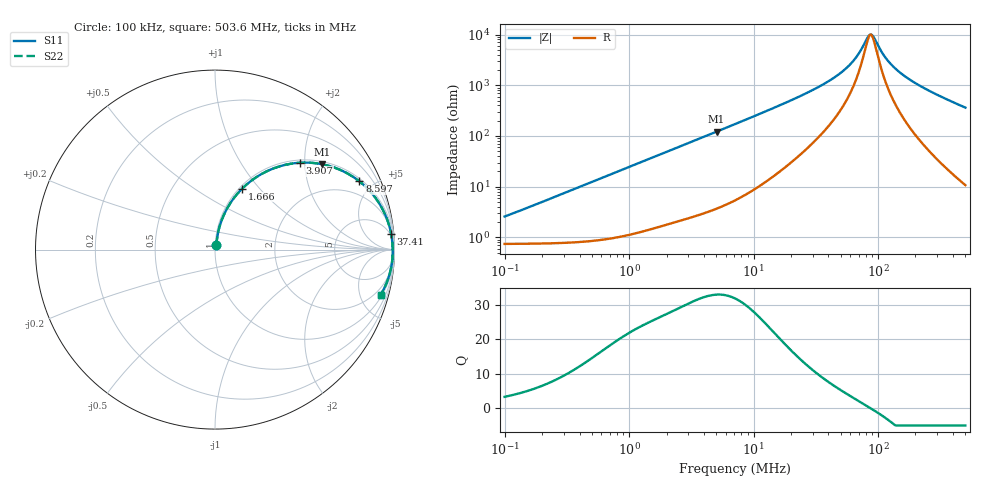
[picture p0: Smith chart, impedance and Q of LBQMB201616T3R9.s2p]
! LBQMB201616T3R9  S-PARAMETER MODEL  ( General Type )
! Model Generated by TAIYO YUDEN Corporation (http://www.ty-top.com)
! Version 1.0
! TAIYO YUDEN Control No. 191025NI43SB-FBB
! Copyright(c) 2019 TAIYO YUDEN CO.,LTD. All Rights Reserved.
! Product Description (link to TY-COMPAS)
! https://ds.yuden.co.jp/TYCOMPAS/or/detail?pn=LBQMB201616T3R9J&u=M
! Products Name : Inductors
! Characteristics :
!  Inductance : 3.9 uH , SRF(min) : 43 MHz , DC Resistance(max) : 0.962 Ohm , Rated Current : 275 mA
!  Case Size : 2.0 x 1.6 / 0.079 x 0.063 [mm/inch] , Thickness : 1.6 / 0.063 [mm/inch]
!  (Conditions: Temperature = 25 degC , DC Bias Current/Voltage = 0A / 0V)
! External Node Assignments :
!  1  o---GGG---o  2
! GND o---------o GND
! Frequency Range : 0.1MHz  -  503.601575MHz  [ 402 STEP ]
# MHz S RI R 50
! Freq[MHz].  S11 Real  S11 Imag  S21 Real  S21 Imag  S12 Real  S12 Imag  S22 Real  S22 Imag
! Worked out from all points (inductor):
!   401 points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, 100 kHz to 503.6 MHz, reference 50 ohm
!   read as one part in series: L = 3.94 uH near 104.4 kHz
!   highest Q = 33 at 5.046 MHz (marker M1), where L = 3.84 uH
!   self-resonance near 85.88 MHz
!   S11 on the Smith chart (normalised r, x): 100 kHz: 1.01, +0.05; 1.666 MHz: 1.03, +0.81; 3.907 MHz: 1.06, +1.89; 8.597 MHz: 1.14, +4.16; 37.41 MHz: 4, +22; 503.6 MHz: 1.21, -7.25
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0.1  0.00799 0.0244  0.992 -0.0244  0.992 -0.0244  0.00799 0.0244
0.416965  0.0184 0.1003  0.9816 -0.1003  0.9816 -0.1003  0.0184 0.1003
0.937126  0.0596 0.2145  0.9404 -0.2145  0.9404 -0.2145  0.0596 0.2145
1.666053  0.1516 0.3399  0.8484 -0.3399  0.8484 -0.3399  0.1516 0.3399
1.738598  0.162 0.3499  0.838 -0.3499  0.838 -0.3499  0.162 0.3499
3.907486  0.4723 0.4839  0.5277 -0.4839  0.5277 -0.4839  0.4723 0.4839
5.046149  0.5947 0.476  0.4053 -0.476  0.4053 -0.476  0.5947 0.476
7.249345  0.7477 0.4189  0.2523 -0.4189  0.2523 -0.4189  0.7477 0.4189
8.596873  0.8048 0.3801  0.1952 -0.3801  0.1952 -0.3801  0.8048 0.3801
14.64606  0.9189 0.2512  0.0811 -0.2512  0.0811 -0.2512  0.9189 0.2512
29.58987  0.9741 0.1204  0.0259 -0.1204  0.0259 -0.1204  0.9741 0.1204
37.4068  0.9812 0.0886  0.0188 -0.0886  0.0188 -0.0886  0.9812 0.0886
48.30734  0.986 0.0587  0.014 -0.0587  0.014 -0.0587  0.986 0.0587
59.78129  0.9883 0.0364  0.0117 -0.0364  0.0117 -0.0364  0.9883 0.0364
69.39878  0.9894 0.0218  0.0106 -0.0218  0.0106 -0.0218  0.9894 0.0218
85.88237  0.9901 0.00155  0.00988 -0.00155  0.00988 -0.00155  0.9901 0.00155
91.55239  0.9902 -0.0045  0.0098 0.0045  0.0098 0.0045  0.9902 -0.0045
108.5704  0.99 -0.0208  0.00996 0.0208  0.00996 0.0208  0.99 -0.0208
123.3794  0.9896 -0.0335  0.0104 0.0335  0.0104 0.0335  0.9896 -0.0335
152.6845  0.9879 -0.056  0.0121 0.056  0.0121 0.056  0.9879 -0.056
205.7633  0.9829 -0.092  0.0171 0.092  0.0171 0.092  0.9829 -0.092
503.6016  0.923 -0.2522  0.077 0.2522  0.077 0.2522  0.923 -0.2522
